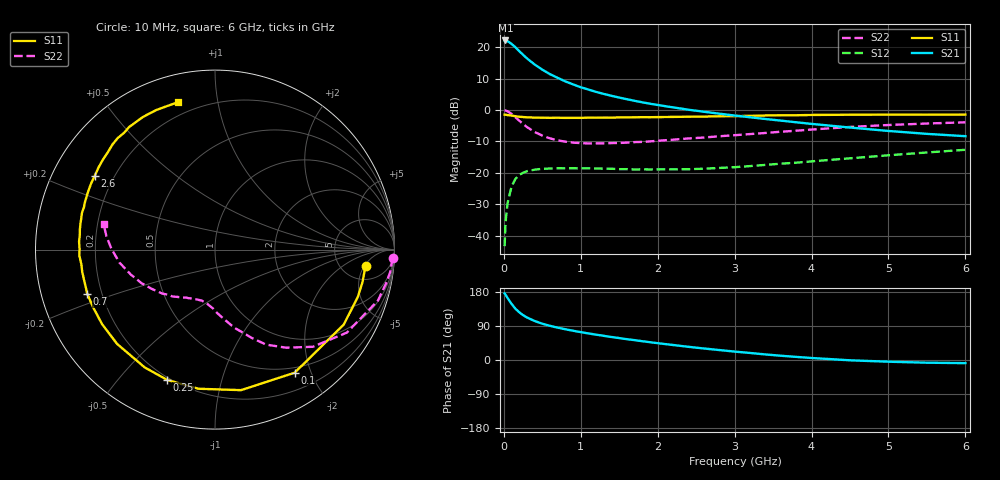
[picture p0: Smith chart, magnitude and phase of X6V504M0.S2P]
! SIEMENS Small Signal Semiconductors
! BFP193W
! Si NPN RF Bipolar Junction Transistor in SOT343
! VCE = 0.5 V  IC = 4 mA
! Common Emitter S-Parameters:  April 1994
# GHz  S  MA  R  50
!  f  S11  S21  S12  S22
! GHz  MAG  ANG  MAG  ANG  MAG  ANG  MAG  ANG
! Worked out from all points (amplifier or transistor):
!   40 points, 10 MHz to 6 GHz, reference 50 ohm
!   highest |S21| = 22.1 dB at 20 MHz (marker M1)
!   |S21| within 3 dB of that: start of sweep to 183.7 MHz
!   unconditionally stable (mu >= 1): 1.641 GHz to end of sweep
!   at 200 MHz: K = 0.14, MSG = 19.7 dB, |S12| = -20.7 dB
!   at 1.5 GHz: K = 0.93, MSG = 11.4 dB, |S12| = -18.8 dB
!   at 6 GHz: K = 1.15, MAG = -0.2 dB, |S12| = -12.7 dB
!   S11 on the Smith chart (normalised r, x): 10 MHz: 8.47, -5.27; 100 MHz: 0.43, -1.76; 250 MHz: 0.19, -0.68; 700 MHz: 0.14, -0.16; 2.6 GHz: 0.13, +0.28; 6 GHz: 0.13, +0.77
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0.01  0.8435 -6.1  12.78 175.8  0.0068 86.7  0.9905 -2.7
0.02  0.8416 -12.3  12.79 173.1  0.0142 82.8  0.9843 -7.2
0.03  0.8383 -18.3  12.73 169.9  0.0206 80.3  0.9737 -10.7
0.05  0.8301 -30.2  12.44 163.1  0.0335 74.2  0.951 -17.4
0.1  0.8169 -57.1  11.29 148.1  0.0605 60.5  0.868 -32.2
0.15  0.7964 -79.5  9.973 135.5  0.0798 49.5  0.7683 -44.8
0.2  0.7807 -96.8  8.646 125.9  0.0924 41.7  0.6758 -54.0
0.25  0.7734 -110.1  7.574 118.4  0.1005 35.4  0.6012 -61.7
0.3  0.7644 -120.8  6.641 112.3  0.1061 30.9  0.5353 -67.2
0.4  0.7574 -136.1  5.306 102.9  0.1123 24.2  0.4472 -76.2
0.5  0.7538 -146.7  4.383 95.8  0.1158 20.2  0.3915 -82.5
0.6  0.7513 -154.8  3.718 90.1  0.117 17.1  0.3538 -88.0
0.7  0.7532 -160.9  3.249 85.4  0.1182 15.3  0.3284 -91.9
0.9  0.7502 -170.2  2.555 77.2  0.1182 12.7  0.3023 -99.0
1.1  0.7563 -177.3  2.114 70.1  0.1179 11.4  0.2932 -104.5
1.6  0.7635 169.1  1.485 54.9  0.1144 11.8  0.3021 -116.0
2.2  0.7762 156.2  1.101 39.6  0.1135 16.3  0.3367 -128.5
2.6  0.786 148.4  0.938 30.4  0.1162 20.6  0.3647 -136.6
3.2  0.8065 137.8  0.766 18.6  0.128 26.3  0.4139 -148.0
4.5  0.841 118.5  0.526 -0.8  0.1703 30.8  0.5374 -172.3
5.5  0.8429 108.7  0.417 -7.1  0.2109 28.8  0.6094 173.0
6  0.8468 104.1  0.383 -8.3  0.2328 27.1  0.6369 167.1
